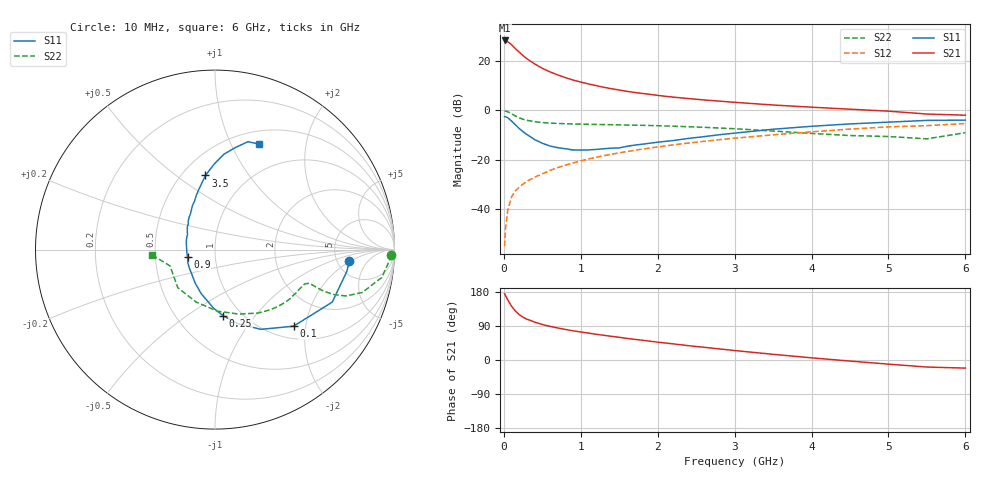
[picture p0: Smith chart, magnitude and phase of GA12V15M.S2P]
! Infineon Technologies  Discrete & RF Semiconductors
! BF775
! Si NPN RF Bipolar Junction Transistor in SOT23
! VCE = 12 V  IC = 15 mA
! Common Emitter S-Parameters:  May  1996
# GHz  S  MA  R  50
!  f  S11  S21  S12  S22
! GHz  MAG  ANG  MAG  ANG  MAG  ANG  MAG  ANG
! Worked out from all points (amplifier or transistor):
!   36 points, 10 MHz to 6 GHz, reference 50 ohm
!   highest |S21| = 28.3 dB at 10 MHz (marker M1)
!   |S21| within 3 dB of that: start of sweep to 140.9 MHz
!   unconditionally stable (mu >= 1): 528.1 MHz to 2.647 GHz
!   at 250 MHz: K = 0.74, MSG = 26.0 dB, |S12| = -29.8 dB
!   at 1.4 GHz: K = 1.09, MAG = 11.4 dB, |S12| = -17.7 dB
!   at 6 GHz: K = 0.86, MSG = 1.7 dB, |S12| = -5.3 dB
!   S11 on the Smith chart (normalised r, x): 10 MHz: 6.50, -1.88; 100 MHz: 1.26, -1.71; 250 MHz: 0.82, -0.70; 900 MHz: 0.73, -0.06; 3.5 GHz: 0.65, +0.65; 6 GHz: 0.65, +1.29
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0.01  0.7516 -4.8  26.01 174.8  0.0018 87.7  0.9831 -1.8
0.02  0.7444 -9.4  25.42 170.8  0.0039 83.7  0.9715 -4.0
0.05  0.716 -24.1  24.58 159.0  0.0094 77.6  0.9422 -9.5
0.1  0.6112 -44.3  21.4 142.2  0.0179 71.5  0.8551 -16.2
0.15  0.5125 -60.1  17.81 129.1  0.0237 65.9  0.7738 -19.5
0.2  0.4306 -73.0  15.1 119.8  0.0282 65.2  0.71 -20.7
0.25  0.3713 -83.0  12.83 112.9  0.0324 64.6  0.6624 -20.9
0.3  0.3261 -91.5  11.1 107.7  0.0368 65.5  0.6324 -20.8
0.4  0.2575 -107.3  8.728 100.1  0.0447 66.2  0.5926 -20.2
0.5  0.2169 -120.6  7.107 93.6  0.0522 67.4  0.5679 -19.8
0.6  0.1909 -131.8  6.021 88.8  0.0613 68.2  0.555 -19.8
0.7  0.1765 -144.0  5.233 84.5  0.0698 68.7  0.5458 -20.3
0.9  0.1584 -164.9  4.117 77.1  0.0868 68.4  0.5325 -21.5
1.1  0.1589 175.9  3.438 71.0  0.1044 68.1  0.5246 -23.6
1.3  0.1682 161.4  2.939 65.2  0.1215 67.1  0.5174 -25.8
1.6  0.188 145.3  2.436 57.0  0.1473 65.1  0.5064 -29.8
2.2  0.2462 123.2  1.859 42.6  0.201 60.5  0.4804 -39.5
2.8  0.3224 108.6  1.544 29.3  0.2561 55.0  0.4409 -51.3
3.5  0.4167 97.3  1.288 15.0  0.3212 47.4  0.3832 -69.7
4.5  0.5341 84.6  1.06 -2.8  0.4196 35.6  0.3107 -109.7
5.5  0.6288 73.0  0.846 -18.6  0.4923 20.1  0.2666 -160.1
6  0.6372 67.2  0.801 -21.4  0.544 15.9  0.3546 -175.4
